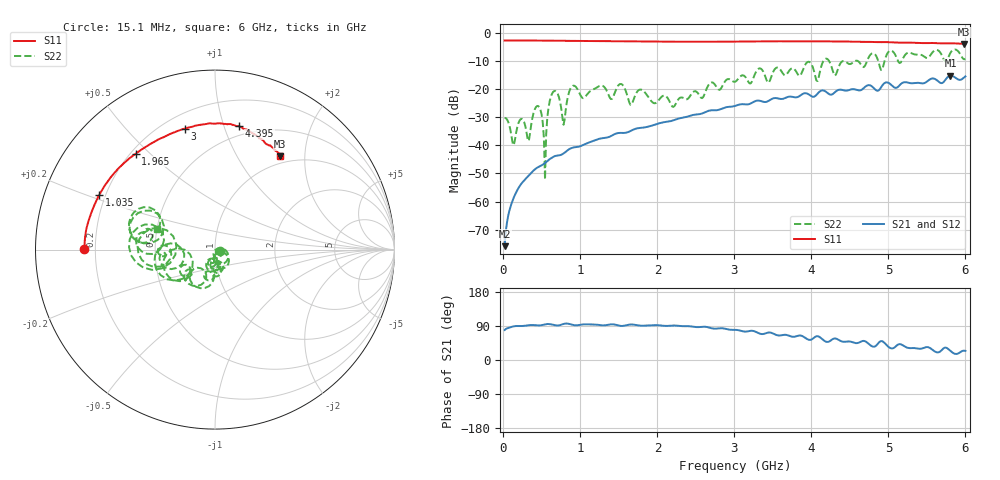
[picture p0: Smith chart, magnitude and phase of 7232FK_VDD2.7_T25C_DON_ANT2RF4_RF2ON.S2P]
!Agilent Technologies,E5071C,MY46417908,A.11.23
!Date: Fri Mar 03 11:29:24 2017
!Data & Calibration Information:
!Freq	S11:SOLT2(ON)	S21:SOLT2(ON)	S12:SOLT2(ON)	S22:SOLT2(ON)
!PortZ  Port1:50+j0  Port2:50+j0
!Above PortZ is port z conversion or system Z0 setting when saving the data.
!When reading, reference impedance value at option line is always used.
# Hz S dB R 50
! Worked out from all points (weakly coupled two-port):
!   400 points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, 15.1 MHz to 6 GHz, reference 50 ohm
!   highest |S21| = -15.29 dB at 5.805 GHz (marker M1); lowest = -75.8 dB at 15.1 MHz (marker M2)
!   lowest |S11| = -4.0 dB at 5.985 GHz (marker M3), VSWR 4.46, Z = 44.2 + j76.9 ohm
!   |S11| at or under -10 dB: nowhere
!   |S22| runs from -52.2 to -6.0 dB; largest |S21 - S12| = 0.0032
!   S11 on the Smith chart (normalised r, x): 15.1 MHz: 0.16, +0.00; 1.035 GHz: 0.18, +0.22; 1.965 GHz: 0.22, +0.45; 3 GHz: 0.28, +0.74; 4.395 GHz: 0.42, +1.12; 6 GHz: 0.88, +1.54
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1.509975e7  -2.76 179.6  -75.84 79.2  -75.86 80.7  -30.25 -9.5
1.050982e8  -2.77 177.6  -60.66 87.4  -60.67 87.3  -36.76 -58.7
3.300945e8  -2.78 172.6  -50.69 91.9  -50.68 91.9  -38.44 -34.9
4.650922e8  -2.80 169.7  -47.55 91.2  -47.55 91.2  -26.42 -78.9
5.100915e8  -2.81 168.7  -46.89 92.6  -46.88 92.7  -31.80 -110.0
5.40091e8  -2.81 167.9  -46.29 93.9  -46.31 94.0  -52.20 -36.6
5.700905e8  -2.82 167.2  -45.65 95.0  -45.65 95.0  -30.06 15.7
6.300895e8  -2.84 165.7  -44.37 93.7  -44.38 93.7  -21.72 -25.0
7.80087e8  -2.88 161.8  -42.91 95.1  -42.93 95.1  -32.71 -64.2
8.850852e8  -2.91 158.9  -40.97 93.5  -40.97 93.5  -19.22 -47.6
1.020083e9  -2.93 155.2  -40.09 93.6  -40.10 93.5  -23.03 -79.8
1.035083e9  -2.93 154.8  -39.90 93.9  -39.92 93.8  -23.27 -75.4
1.965067e9  -3.18 129.5  -32.70 92.0  -32.71 92.0  -25.08 -103.0
2.010066e9  -3.19 128.3  -32.29 91.7  -32.30 91.8  -24.18 -93.9
3.00005e9  -3.16 104.0  -26.08 79.7  -26.08 79.8  -17.46 -94.3
3.01505e9  -3.16 103.7  -25.96 79.6  -25.95 79.7  -17.35 -92.6
4.005033e9  -3.07 84.7  -22.64 54.5  -22.62 54.4  -11.39 -174.9
4.395027e9  -3.09 79.0  -20.30 49.0  -20.29 49.0  -10.29 -163.2
5.010016e9  -3.37 70.8  -17.95 33.3  -17.89 33.4  -6.58 -176.2
5.805003e9  -3.76 58.8  -15.29 24.1  -15.26 24.8  -7.18 173.4
5.985e9  -3.96 55.1  -15.86 24.7  -15.88 25.3  -9.47 156.2
6e9  -3.95 55.1  -15.53 24.1  -15.54 24.9  -9.28 160.7
